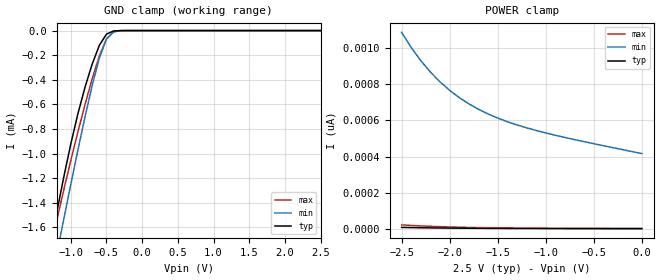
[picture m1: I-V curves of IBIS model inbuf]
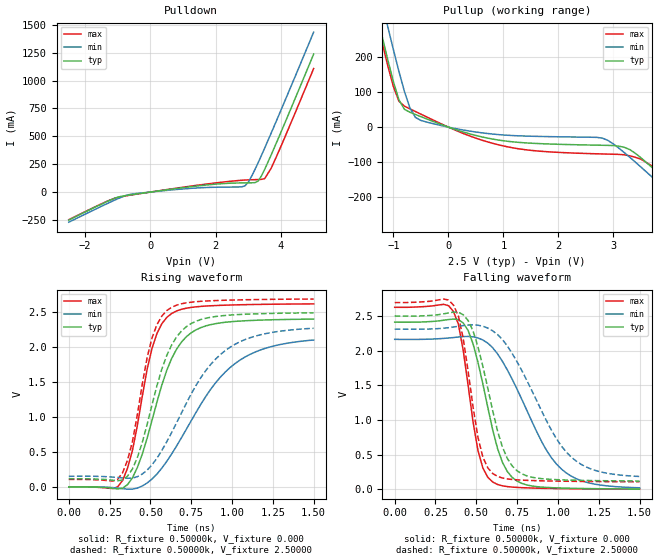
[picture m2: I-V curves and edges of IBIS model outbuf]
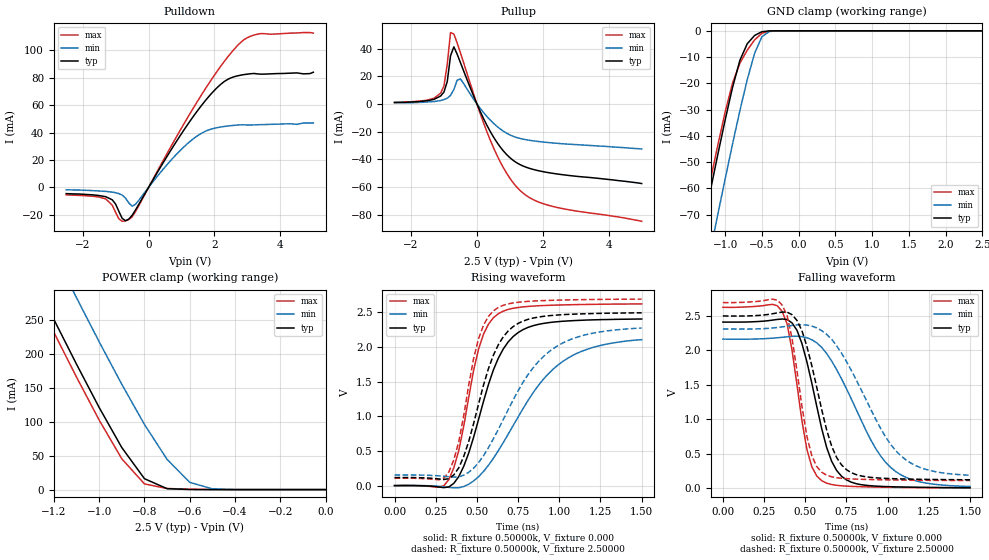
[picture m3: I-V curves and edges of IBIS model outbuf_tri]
| IBIS file 49fct208.ibs created by s2ibis2 version 1.2
| North Carolina State University Electronics Research Laboratory  1995
[IBIS ver]   2.1
[File name]   49fct208.ibs
[File Rev]   0.1
[Date]   04/24/2003 smg
[Source]   Integrated Device Technology, Inc.
[Notes]   1.Temperatures: typ=25C, min=150C, max=0C
[Disclaimer] Integrated Device Technology, Inc. ("IDT") hereby grants the
   user of this IBIS model a non-exclusive, nontransferable
   license to use this IBIS model under the following terms. The
   user is granted this license only to use the IBIS model and is
   not granted rights to sell, copy (except as needed to run the
   IBIS model), rent, lease or sub-license the IBIS model in
   whole or in part, or in modified form to anyone. The User may
   modify the IBIS model to suit its specific applications, but
   rights to derivative works and such modifications shall belong
   to IDT. This IBIS model is provided on an AS IS" basis and IDT
   makes absolutely no warranty with respect to the information
   contained herein. IDT DISCLAIMS AND CUSTOMER WAIVES ALL
   WARRANTIES, EXPRESS AND IMPLIED, INCLUDING WARRANTIES OF
   MERCHANTABILITY AND FITNESS FOR A PARTICULAR PURPOSE. THE
   ENTIRE RISK AS TO QUALITY AND PERFORMANCE IS WITH THE USER
   ACCORDINGLY, IN NO EVENT SHALL IDT BE LIABLE FOR ANY DIRECT OR
   INDIRECT DAMAGES, WHETHER IN CONTRACT OR TORT, INCLUDING ANY
   LOST PROFITS OR OTHER INCIDENTAL, CONSEQUENTIAL, EXEMPLARY, OR
   PUNITIVE DAMAGES ARISING OUT OF THE USE OR APPLICATION OF THE
   IBIS model. Further, IDT reserves the right to make changes
   without notice to any product herein to improve reliability,
   function, or design. IDT does not convey any license under
   patent rights or any other intellectual property rights,
   including those of third parties. IDT is not obligated to
   provide maintenance or support for the licensed IBIS model.
[Copyright]   Copyright 1997, Integrated Device Technology, Inc. all rights
   reserved
|   Component 49fct20805
[Component]   49fct20805
[Manufacturer]   Integrated Device Technology, Inc.
[Package]
| variable   typ   min   max
R_pkg   60.00000m   50.00000m   90.00000m
L_pkg   2.50000nH   1.50000nH   3.00000nH
C_pkg   0.14000pF   0.10000pF   0.18000pF
[Pin]  signal_name   model_name   R_pin   L_pin   C_pin
1   VCCA   POWER
2   OA1   outbuf_tri
3   OA2   outbuf_tri
4   OA3   outbuf_tri
5   GNDA   GND
6   OA4   outbuf_tri
7   OA5   outbuf_tri
8   GNDQ   GND
9   OEAB   inbuf
10   INA   inbuf
11   INB   inbuf
12   OEBB   inbuf
13   MON   outbuf
14   OB5   outbuf_tri
15   OB4   outbuf_tri
16   GNDB   GND
17   OB3   outbuf_tri
18   OB2   outbuf_tri
19   OB1   outbuf_tri
20   VCCB   POWER
| Models and submodels in the file (3): inbuf (Input), outbuf (Output), outbuf_tri (3-state)
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|   Model inbuf
[Model]   inbuf
Model_type   Input
Polarity   Inverting
Vinl =  0.70000V
Vinh =  1.70000V
Vmeas =  1.25000V
C_comp   2.60000pF   NA   NA
[Temperature Range]   25.00000   0.15000k   0.000
[Voltage Range]   2.50000V   2.30000V   2.70000V
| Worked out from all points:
|   GND clamp passes 1 mA (typ) near -1.03 V on its own axis
[GND_clamp]
| voltage   I(typ)   I(min)   I(max)
-2.5V     -5.693mA   -5.744mA   -5.655mA
-1.3V     -1.792mA   -2.121mA   -1.821mA
-1.2V     -1.488mA   -1.827mA   -1.552mA
-1.1V     -1.195mA   -1.537mA   -1.299mA
-900mV    -674.9uA   -969.9uA   -823.3uA
-800mV    -458.9uA   -699.2uA   -600.1uA
-700mV    -271.4uA   -445uA     -391uA
-600mV    -119.9uA   -223.2uA   -205.7uA
-500mV    -28.6uA    -68.61uA   -67.73uA
-400mV    -2.904uA   -10.33uA   -9.139uA
-300mV    -131.8nA   -985.5nA   -473.5nA
2.5V      2.102pA    438.2pA    2.842pA
[POWER_clamp]
| voltage   I(typ)   I(min)   I(max)
-2.5V     9.124pA    1.085nA    22.79pA
-2.4V     8.098pA    1.001nA    19.81pA
-2.3V     7.135pA    928.7pA    17.3pA
-2.2V     6.403pA    865.8pA    15.03pA
-2.1V     5.793pA    811.8pA    13.06pA
-2V       5.185pA    765.3pA    11.5pA
-1.9V     4.749pA    725.2pA    10.12pA
-1.7V     4.004pA    660.9pA    7.891pA
-1.4V     3.3pA      592.4pA    5.761pA
-1.1V     2.86pA     543.9pA    4.466pA
-700mV    2.494pA    493.5pA    3.654pA
0V        2.103pA    416.7pA    2.908pA
|   Model outbuf
[Model]   outbuf
Model_type   Output
Polarity   Non-Inverting
Vmeas =  1.25000V
C_comp   5.50000pF   NA   NA
[Temperature Range]   25.00000   0.15000k   0.000
[Voltage Range]   2.50000V   2.30000V   2.70000V
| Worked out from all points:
|   slope of the pulldown table from 0 to 0.375 V, typ, clamps not added: 24.5 ohm
|   slope of the pullup table from 0 to 0.375 V, typ, clamps not added: 20.1 ohm
|   rising waveform, R_fixture 0.50000k, V_fixture 0.000: 20-80 % time 197ps typ, 360ps min, 136ps max; typ from 0 V to 2.4 V
|   rising waveform, R_fixture 0.50000k, V_fixture 2.50000: 20-80 % time 183ps typ, 324ps min, 129ps max; typ from 0.116 V to 2.49 V
|   falling waveform, R_fixture 0.50000k, V_fixture 0.000: 20-80 % time 146ps typ, 275ps min, 102ps max; typ from 2.41 V to 0.005 V
|   falling waveform, R_fixture 0.50000k, V_fixture 2.50000: 20-80 % time 149ps typ, 288ps min, 104ps max; typ from 2.5 V to 0.121 V
[Pulldown]
| voltage   I(typ)   I(min)   I(max)
-2.5V     -251.1mA   -270.4mA   -247.9mA
-1.3V     -81.22mA   -100.3mA   -78.79mA
-1V       -46.01mA   -60.14mA   -49.02mA
-600mV    -24.86mA   -19.87mA   -26.91mA
1.6V      59.57mA    39.41mA    67.25mA
2.9V      82.28mA    56.29mA    107.8mA
3.1V      83.07mA    141.5mA    110.3mA
3.3V      98.88mA    263.5mA    112.2mA
3.5V      203.6mA    394.7mA    120.5mA
3.7V      333.6mA    529.7mA    214.2mA
4.1V      607.1mA    805mA      479.5mA
5V        1.238A     1.435A     1.108A
[Pullup]
| voltage   I(typ)   I(min)   I(max)
-2.5V     1.155A     1.248A     1.137A
-1.3V     321.4mA    417.7mA    303.2mA
-1.1V     190.5mA    285.1mA    173.6mA
-900mV    78.05mA    159.2mA    74.08mA
-800mV    50.9mA     102.1mA    59.98mA
-500mV    29.9mA     19.1mA     37.05mA
1V        -38.88mA   -22.4mA    -53.74mA
2.8V      -51.78mA   -31.39mA   -76.61mA
3.3V      -64.2mA    -86.17mA   -81.91mA
3.7V      -114.5mA   -141.9mA   -110.5mA
4.7V      -259.7mA   -286.4mA   -253.5mA
5V        -304.2mA   -330.3mA   -298.3mA
[Ramp]
| variable   typ   min   max
dV/dt_r   1.01400/0.21661n   0.68520/0.37207n   1.21140/0.14535n
dV/dt_f   0.99528/0.15774n   0.78066/0.33704n   1.10952/0.10279n
R_load = 50.00000
[Rising Waveform]
R_fixture = 0.50000k
V_fixture = 0.000
L_fixture = 0.000H
| time   V(typ)   V(min)   V(max)
0s        189.5uV    183.9uV    227.6uV
270ps     -20.5mV    -10.08mV   -23.55mV
330ps     -18.09mV   -25.22mV   94.05mV
390ps     130.3mV    -32.24mV   522.9mV
510ps     954.6mV    113.3mV    1.986V
570ps     1.46V      268.7mV    2.337V
630ps     1.839V     471.8mV    2.483V
780ps     2.251V     1.069V     2.579V
1.02ns    2.372V     1.77V      2.607V
1.5ns     2.404V     2.104V     2.622V
[Rising Waveform]
R_fixture = 0.50000k
V_fixture = 2.50000
L_fixture = 0.000H
| time   V(typ)   V(min)   V(max)
0s        115.5mV    152mV      107.1mV
270ps     95.78mV    141.1mV    84.43mV
330ps     100.7mV    128mV      204.2mV
390ps     257.4mV    126.2mV    649.5mV
420ps     419.8mV    146.6mV    1.034V
510ps     1.177V     315.8mV    2.135V
600ps     1.882V     646.2mV    2.525V
720ps     2.295V     1.198V     2.637V
960ps     2.457V     1.956V     2.675V
1.5ns     2.493V     2.272V     2.691V
[Falling Waveform]
R_fixture = 0.50000k
V_fixture = 0.000
L_fixture = 0.000H
| time   V(typ)   V(min)   V(max)
0s        2.41V      2.163V     2.624V
360ps     2.455V     2.189V     2.565V
420ps     2.398V     2.203V     2.002V
510ps     1.833V     2.183V     562mV
600ps     862.1mV    2.043V     107mV
660ps     390.4mV    1.845V     51.81mV
720ps     172.7mV    1.587V     33.55mV
900ps     33.57mV    689.3mV    16.5mV
1.02ns    19.95mV    296.3mV    11.56mV
1.5ns     5.368mV    23.54mV    3.544mV
[Falling Waveform]
R_fixture = 0.50000k
V_fixture = 2.50000
L_fixture = 0.000H
| time   V(typ)   V(min)   V(max)
0s        2.499V     2.311V     2.693V
360ps     2.555V     2.341V     2.657V
420ps     2.517V     2.361V     2.172V
480ps     2.285V     2.373V     1.188V
540ps     1.776V     2.352V     467.4mV
600ps     1.138V     2.286V     230.2mV
690ps     446mV      2.067V     151.2mV
780ps     223.1mV    1.707V     133.6mV
1.08ns    133.4mV    469.4mV    116.8mV
1.5ns     120.9mV    186.7mV    110.4mV
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|   Model outbuf_tri
[Model]   outbuf_tri
Model_type   3-state
Polarity   Non-Inverting
Enable   Active-High
Vmeas =  1.25000V
C_comp   5.50000pF   NA   NA
[Temperature Range]   25.00000   0.15000k   0.000
[Voltage Range]   2.50000V   2.30000V   2.70000V
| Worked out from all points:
|   slope of the pulldown table from 0 to 0.375 V, typ, clamps not added: 24.5 ohm
|   slope of the pullup table from 0 to 0.375 V, typ, clamps not added: 20.1 ohm
|   GND clamp passes 1 mA (typ) near -0.55 V on its own axis
|   POWER clamp passes 1 mA (typ) near -0.67 V on its own axis
|   rising waveform, R_fixture 0.50000k, V_fixture 0.000: 20-80 % time 197ps typ, 358ps min, 136ps max; typ from 0 V to 2.4 V
|   rising waveform, R_fixture 0.50000k, V_fixture 2.50000: 20-80 % time 183ps typ, 321ps min, 129ps max; typ from 0.116 V to 2.49 V
|   falling waveform, R_fixture 0.50000k, V_fixture 0.000: 20-80 % time 146ps typ, 275ps min, 102ps max; typ from 2.41 V to 0.005 V
|   falling waveform, R_fixture 0.50000k, V_fixture 2.50000: 20-80 % time 149ps typ, 288ps min, 104ps max; typ from 2.5 V to 0.121 V
[Pulldown]
| voltage   I(typ)   I(min)   I(max)
-2.5V     -4.5mA     -1.7mA     -5.4mA
-1.3V     -6.75mA    -2.87mA    -8.33mA
-1.1V     -9.05mA    -3.42mA    -13.02mA
-900mV    -17.52mA   -4.48mA    -22.92mA
-800mV    -22.58mA   -5.59mA    -24.68mA
-600mV    -23.1mA    -11.3mA    -23.45mA
-400mV    -16.54mA   -12.36mA   -17.81mA
1.4V      53.17mA    36.22mA    59.5mA
2.2V      75.38mA    44.11mA    88.7mA
2.7V      81.36mA    45.48mA    103.5mA
3.4V      82.58mA    45.8mA     112.1mA
5V        84mA       47mA       112.5mA
[Pullup]
| voltage   I(typ)   I(min)   I(max)
-2.5V     1mA        1mA        1mA
-1.1V     5.7mA      2.4mA      7.8mA
-1V       8.6mA      3.1mA      13mA
-900mV    16.13mA    4.1mA      28.65mA
-800mV    34.8mA     6.14mA     51.58mA
-700mV    41.24mA    10.36mA    50.54mA
-500mV    29.87mA    18.03mA    36.95mA
400mV     -19.74mA   -11.59mA   -25.9mA
900mV     -36.59mA   -21.16mA   -50.06mA
1.3V      -43.8mA    -24.95mA   -62.39mA
2.3V      -50.21mA   -28.24mA   -74.14mA
5V        -57.6mA    -32.6mA    -84.9mA
[GND_clamp]
| voltage   I(typ)   I(min)   I(max)
-2.5V     -246.6mA   -268.7mA   -242.5mA
-1.4V     -88.48mA   -111.4mA   -84.4mA
-1.3V     -74.47mA   -97.43mA   -70.46mA
-1.2V     -60.62mA   -83.55mA   -56.75mA
-1.1V     -47.02mA   -69.82mA   -43.42mA
-900mV    -21.55mA   -43.09mA   -19.88mA
-800mV    -11.23mA   -30.38mA   -12.34mA
-700mV    -4.919mA   -18.57mA   -7.359mA
-600mV    -1.764mA   -8.573mA   -3.458mA
-500mV    -338.8uA   -2.238mA   -928.1uA
-400mV    -30.89uA   -266.5uA   -103.1uA
2.5V      19.02pA    887.4nA    -22.82pA
[POWER_clamp]
| voltage   I(typ)   I(min)   I(max)
-2.5V     1.154A     1.247A     1.136A
-1.3V     318.1mA    416mA      299.1mA
-1.2V     250.8mA    348.9mA    231.8mA
-1.1V     184.8mA    282.7mA    165.8mA
-1V       121mA      217.8mA    102.5mA
-900mV    61.92mA    155.1mA    45.43mA
-800mV    16.1mA     95.96mA    8.399mA
-700mV    1.327mA    44.44mA    1.653mA
-600mV    180.8uA    10.66mA    505uA
-500mV    26.61uA    1.071mA    96.76uA
0V        19.08pA    11.69nA    32.15pA
[Ramp]
| variable   typ   min   max
dV/dt_r   1.01400/0.21662n   0.68640/0.36764n   1.21140/0.14637n
dV/dt_f   0.99528/0.15774n   0.78066/0.33674n   1.10952/0.10273n
R_load = 50.00000
[Rising Waveform]
R_fixture = 0.50000k
V_fixture = 0.000
L_fixture = 0.000H
| time   V(typ)   V(min)   V(max)
0s        189.6uV    183.9uV    227.6uV
330ps     -18.08mV   -25.73mV   88.46mV
390ps     130.4mV    -31.01mV   506.7mV
510ps     954.6mV    128.8mV    1.97V
570ps     1.46V      293.3mV    2.329V
630ps     1.839V     504.6mV    2.481V
750ps     2.208V     989.8mV    2.571V
990ps     2.365V     1.736V     2.606V
1.2ns     2.392V     1.991V     2.615V
1.5ns     2.404V     2.106V     2.622V
[Rising Waveform]
R_fixture = 0.50000k
V_fixture = 2.50000
L_fixture = 0.000H
| time   V(typ)   V(min)   V(max)
0s        115.5mV    152mV      107.1mV
270ps     95.78mV    140.9mV    84.27mV
330ps     100.7mV    127.5mV    198.7mV
390ps     257.5mV    127.4mV    633.2mV
420ps     419.9mV    150.3mV    1.012V
510ps     1.177V     331.7mV    2.12V
600ps     1.882V     675.7mV    2.522V
720ps     2.295V     1.237V     2.636V
960ps     2.457V     1.972V     2.675V
1.5ns     2.493V     2.274V     2.691V
[Falling Waveform]
R_fixture = 0.50000k
V_fixture = 0.000
L_fixture = 0.000H
| time   V(typ)   V(min)   V(max)
0s        2.41V      2.163V     2.624V
360ps     2.455V     2.189V     2.565V
420ps     2.398V     2.203V     2.001V
510ps     1.833V     2.183V     561.7mV
600ps     862.1mV    2.043V     107mV
660ps     390.5mV    1.845V     51.81mV
720ps     172.7mV    1.587V     33.55mV
900ps     33.57mV    689.7mV    16.5mV
1.02ns    19.96mV    296.5mV    11.56mV
1.5ns     5.368mV    23.55mV    3.543mV
[Falling Waveform]
R_fixture = 0.50000k
V_fixture = 2.50000
L_fixture = 0.000H
| time   V(typ)   V(min)   V(max)
0s        2.499V     2.311V     2.693V
360ps     2.555V     2.341V     2.657V
420ps     2.517V     2.361V     2.171V
480ps     2.285V     2.373V     1.187V
540ps     1.776V     2.352V     467.2mV
600ps     1.138V     2.286V     230.1mV
690ps     446mV      2.067V     151.2mV
780ps     223.2mV    1.707V     133.6mV
1.08ns    133.4mV    469.8mV    116.8mV
1.5ns     120.9mV    186.7mV    110.4mV
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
